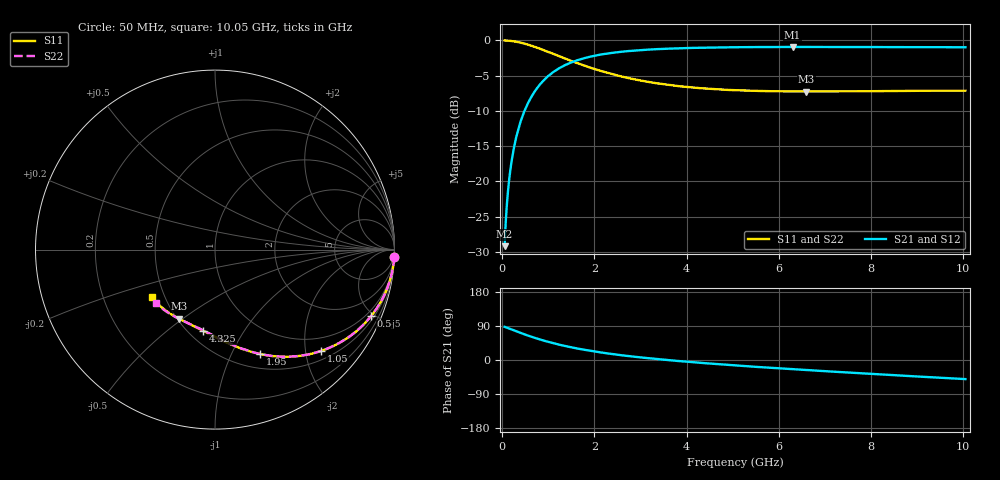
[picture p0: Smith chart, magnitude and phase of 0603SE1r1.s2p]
! AVX Thin Film Operation		Date: August 2001
! Description: Accu-P® Series, Thin Film, SMD, RF Capacitor
! Part Number: 06035J1R1ABT
! 50 MHz  -  10.05 GHz
! Serial Measurements
# mhz S db R 50
!	S11		S21		S12		S22
!	dB	Phase	dB	Phase	dB	Phase	dB	Phase
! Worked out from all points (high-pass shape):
!   401 points, 50 MHz to 10.05 GHz, reference 50 ohm
!   highest |S21| = -0.93 dB at 6.3 GHz (marker M1); lowest = -29.2 dB at 50 MHz (marker M2)
!   |S21| within 3 dB of the highest: 1.24 GHz to end of sweep
!   lowest |S11| = -7.3 dB at 6.6 GHz (marker M3), VSWR 2.53, Z = 25.5 - j24.2 ohm
!   |S11| at or under -10 dB: nowhere
!   |S22| runs from -7.2 to 0.0 dB; largest |S21 - S12| = 0
!   S11 on the Smith chart (normalised r, x): 50 MHz: 1, -48; 500 MHz: 0.69, -4.79; 1.05 GHz: 0.68, -2.32; 1.95 GHz: 0.66, -1.30; 4.325 GHz: 0.59, -0.68; 10.05 GHz: 0.43, -0.28
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50  -0.01 -2.4  -29.20 87.6  -29.20 87.6  -0.01 -2.4
75  -0.01 -3.6  -25.71 86.4  -25.71 86.4  -0.01 -3.6
125  -0.03 -6.0  -21.29 84.0  -21.29 84.0  -0.03 -6.0
150  -0.05 -7.2  -19.71 82.8  -19.71 82.8  -0.05 -7.2
225  -0.10 -10.7  -16.26 79.3  -16.26 79.3  -0.10 -10.7
275  -0.16 -13.1  -14.54 76.9  -14.54 76.9  -0.16 -13.1
350  -0.25 -16.5  -12.59 73.5  -12.59 73.5  -0.25 -16.5
500  -0.49 -23.2  -9.73 66.8  -9.73 66.8  -0.49 -23.2
750  -1.01 -33.3  -6.81 56.7  -6.81 56.7  -1.01 -33.3
1050  -1.76 -43.8  -4.78 46.2  -4.78 46.2  -1.76 -43.8
1375  -2.61 -53.5  -3.46 36.5  -3.46 36.5  -2.61 -53.4
1725  -3.45 -61.9  -2.61 28.1  -2.61 28.1  -3.45 -61.8
1950  -3.95 -66.6  -2.25 23.5  -2.25 23.5  -3.95 -66.4
2625  -5.18 -78.1  -1.58 12.0  -1.58 12.0  -5.18 -77.7
3400  -6.12 -88.2  -1.22 2.0  -1.22 2.0  -6.12 -87.6
4325  -6.79 -98.1  -1.04 -7.7  -1.04 -7.7  -6.78 -97.0
5050  -7.06 -104.6  -0.97 -14.2  -0.97 -14.2  -7.05 -103.6
6300  -7.24 -115.0  -0.93 -24.3  -0.93 -24.3  -7.22 -113.0
6600  -7.25 -117.4  -0.93 -26.6  -0.93 -26.6  -7.23 -115.0
6725  -7.25 -118.9  -0.93 -27.5  -0.93 -27.5  -7.23 -115.9
8400  -7.18 -131.2  -0.95 -39.3  -0.95 -39.3  -7.16 -127.2
10050  -7.13 -142.8  -0.97 -50.4  -0.97 -50.4  -7.09 -137.8
